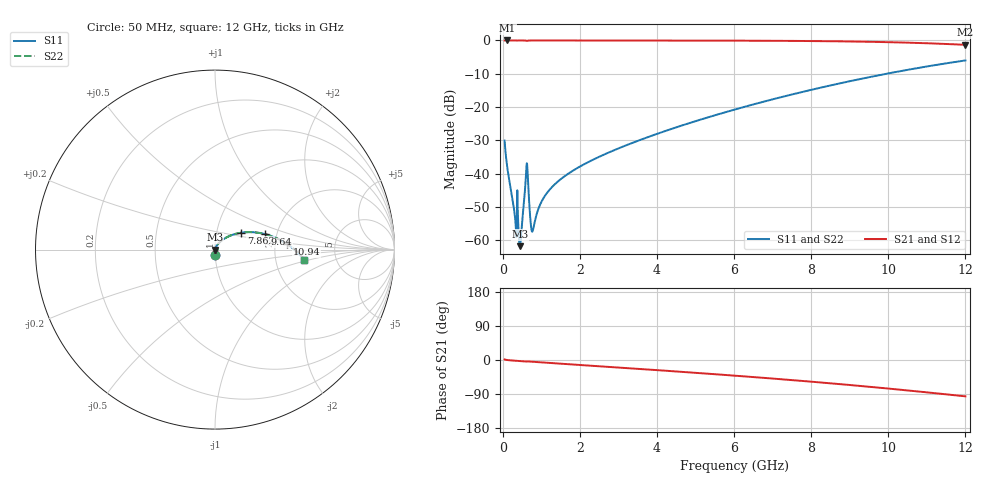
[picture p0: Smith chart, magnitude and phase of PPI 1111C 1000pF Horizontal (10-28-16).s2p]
# MHz S MA R 50
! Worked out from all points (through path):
!   1601 points, 50 MHz to 12 GHz, reference 50 ohm
!   highest |S21| = 0.00 dB at 124.7 MHz (marker M1); lowest = -1.3 dB at 12 GHz (marker M2)
!   group delay of S21, straight-line fit = 21.8 ps
!   lowest |S11| = -61.8 dB at 445.8 MHz (marker M3), VSWR 1.00, Z = 50.1 - j0.00893 ohm
!   |S11| at or under -10 dB: start of sweep to 9.956 GHz
!   |S22| runs from -61.8 to -6.0 dB; largest |S21 - S12| = 0
!   S11 on the Smith chart (normalised r, x): 50 MHz: 1.00, -0.06; 7.862 GHz: 1.31, +0.25; 9.64 GHz: 1.73, +0.33; 10.94 GHz: 2.32, +0.18; 12 GHz: 2.93, -0.44
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50  0.03133 -88.0  0.9992 1.5  0.9992 1.5  0.03133 -88.0
124.6875  0.01177 -88.0  0.9995 -0.1  0.9995 -0.1  0.01177 -88.0
303.9375  0.002667 -77.7  0.9993 -1.7  0.9993 -1.7  0.002667 -77.7
401.0312  0.001891 -63.5  0.9991 -2.4  0.9991 -2.4  0.001891 -63.5
445.8438  0.0008151 -6.3  0.9992 -2.8  0.9992 -2.8  0.0008151 -6.3
490.6562  0.001492 48.6  0.999 -3.1  0.999 -3.1  0.001492 48.6
580.2812  0.005916 60.5  0.9974 -3.9  0.9974 -3.9  0.005916 60.5
617.625  0.01299 28.6  0.989 -4.2  0.989 -4.2  0.01299 28.6
662.4375  0.006644 -47.2  0.9951 -3.9  0.9951 -3.9  0.006644 -47.2
737.125  0.00157 -22.0  0.9985 -4.6  0.9985 -4.6  0.00157 -22.0
781.9375  0.001401 21.8  0.9987 -4.9  0.9987 -4.9  0.001401 21.8
968.6562  0.003408 65.1  0.9988 -6.2  0.9988 -6.2  0.003408 65.1
1177.781  0.005395 70.3  0.9988 -7.6  0.9988 -7.6  0.005395 70.3
2044.156  0.01318 70.5  0.9984 -13.4  0.9984 -13.4  0.01318 70.5
4038.312  0.04023 60.2  0.997 -27.0  0.997 -27.0  0.04023 60.2
6025  0.09197 47.0  0.9928 -41.4  0.9928 -41.4  0.09197 47.0
7862.312  0.1735 32.9  0.981 -56.0  0.981 -56.0  0.1735 32.9
8019.156  0.1823 31.6  0.9793 -57.3  0.9793 -57.3  0.1823 31.6
9639.875  0.2912 17.3  0.9518 -71.9  0.9518 -71.9  0.2912 17.3
10013.31  0.3209 13.7  0.9421 -75.5  0.9421 -75.5  0.3209 13.7
10939.44  0.401 4.6  0.9104 -84.7  0.9104 -84.7  0.401 4.6
12000  0.5008 -6.5  0.8592 -95.9  0.8592 -95.9  0.5008 -6.5
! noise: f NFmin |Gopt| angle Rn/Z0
50  0.0003797  0.8685  0.3291  0.0006214
1372  0.003954  0.6885  8.49  0.002455
2701  0.006443  0.6396  16.55  0.003308
4031  0.008727  0.6172  24.36  0.004066
5360  0.01095  0.6085  31.82  0.004814
6682  0.01319  0.6095  38.86  0.005608
8012  0.01556  0.6178  45.52  0.00651
9341  0.0181  0.6321  51.76  0.007573
1.067e+04  0.0209  0.6513  57.62  0.008868
1.2e+04  0.02407  0.6743  63.13  0.01049
